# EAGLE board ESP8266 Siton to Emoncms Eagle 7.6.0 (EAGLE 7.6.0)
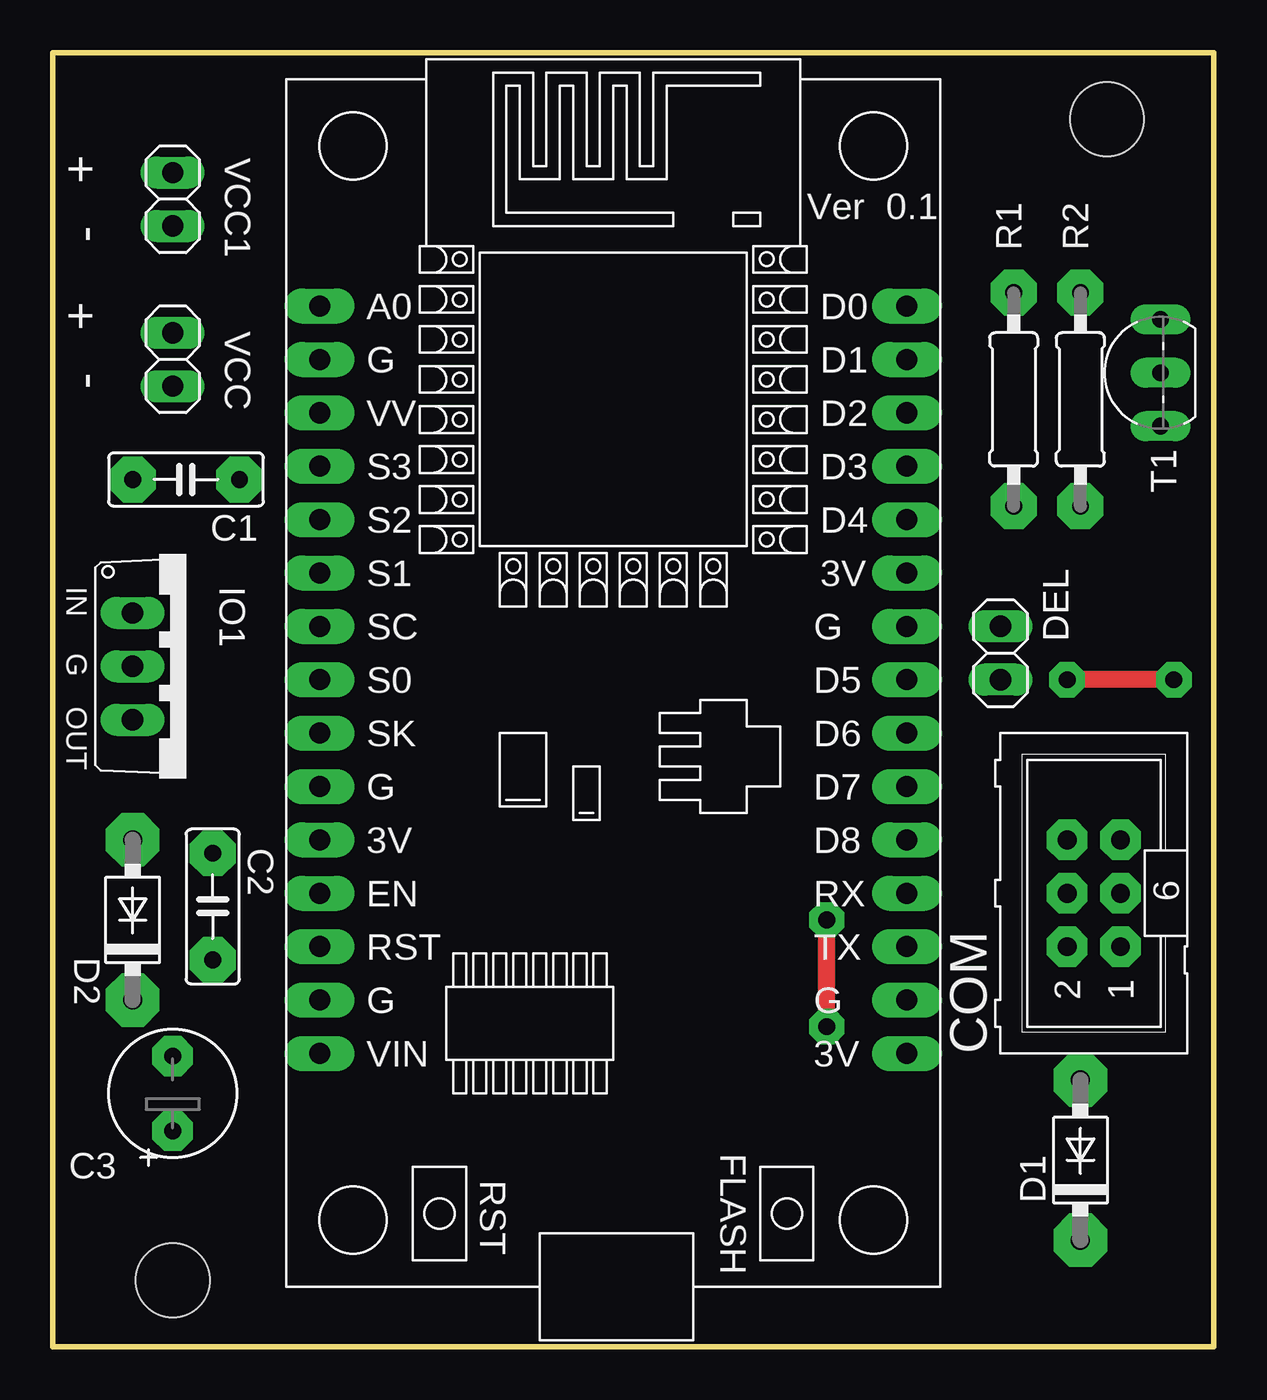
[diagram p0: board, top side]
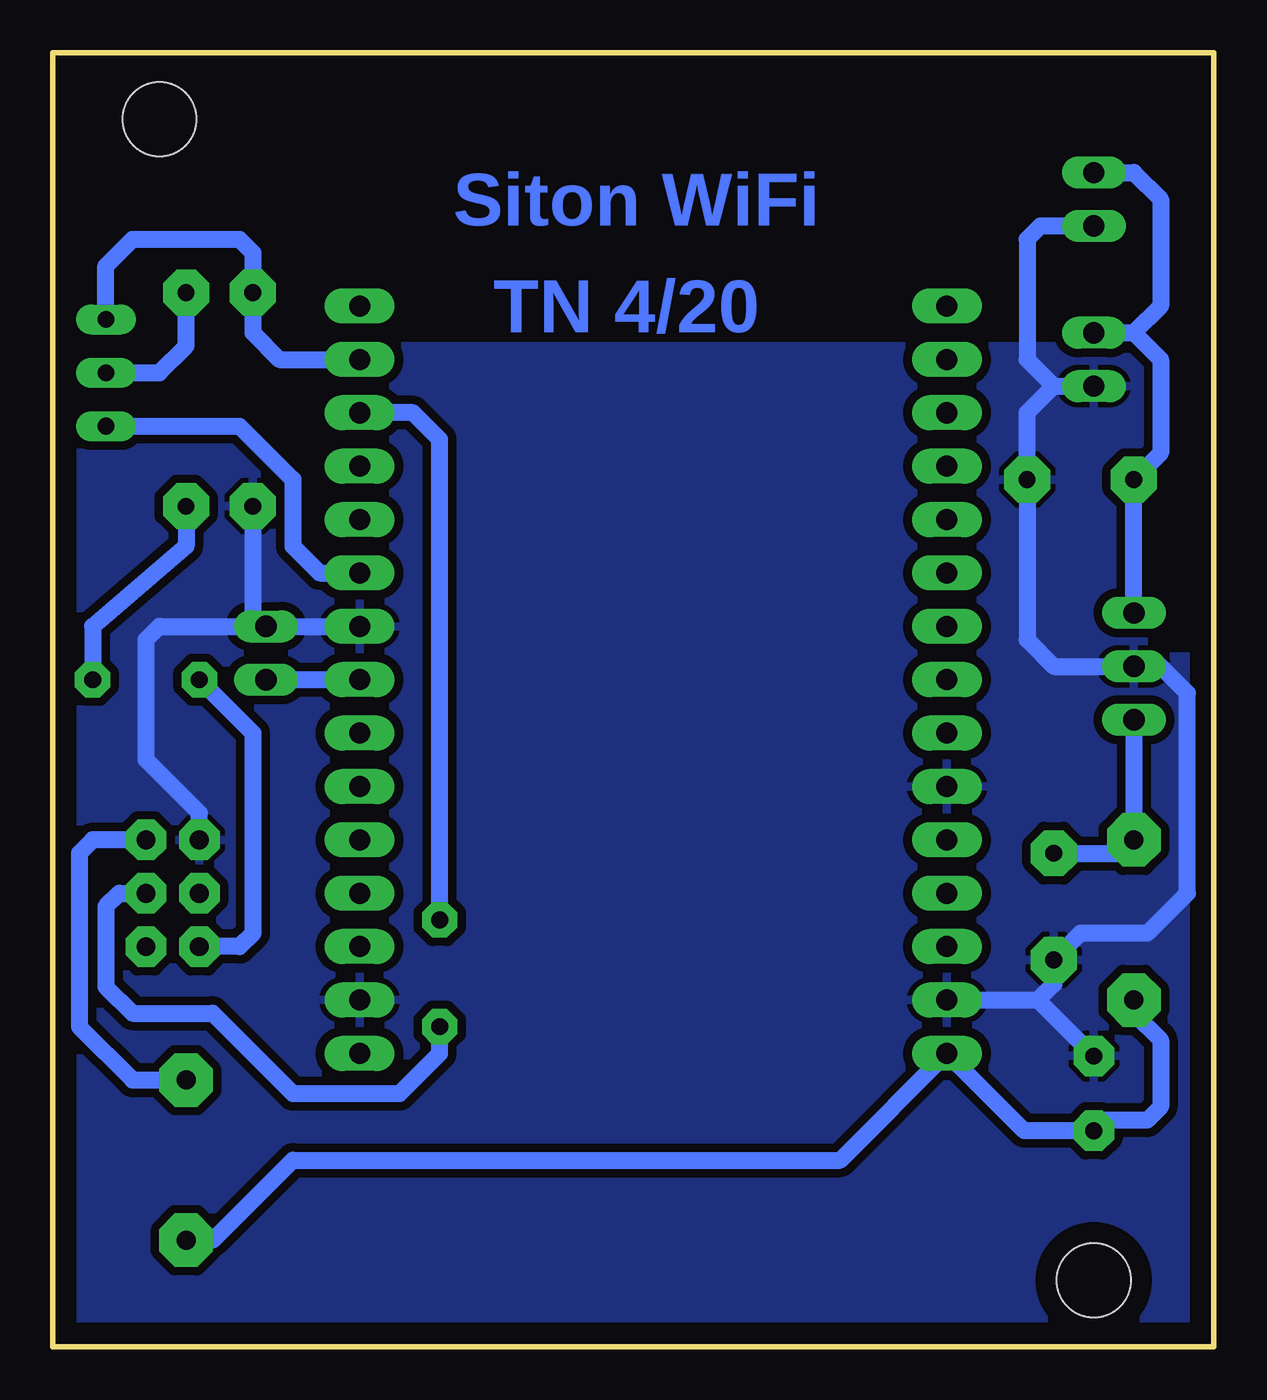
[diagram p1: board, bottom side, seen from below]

Size 55.24 x 61.59 mm. Coordinates in mm from the lower left corner, seen from the top.
Outline: 0,0 55.24,0 55.24,61.59 0,61.59 0,0
Copper layers (1*16): Top 0.035mm / dielectric 1.5mm / Bottom 0.035mm
Design rules "default": minimum track width 10mil, minimum drill 24mil, track to track 8mil, track to pad 8mil, pad to pad 8mil, via to via 8mil, smd to smd 8mil, copper to edge 40mil, drill to drill 8mil, minimum pad ring 10mil, minimum via ring 8mil, stop-mask expansion 4mil, vias tented up to drill 0mil, thermal gap 10mil
Holes 3.5 mm at 50.16,58.42 5.71,3.17
bRestrict: area 0,33.7 to 2.5,51.4

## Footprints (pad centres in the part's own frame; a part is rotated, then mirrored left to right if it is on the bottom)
C050-025X075 = drill 0.8 pad 2.184 octagon: 1 -2.54,0; 2 2.54,0
E3,5-8 = drill 0.8 pad 1.93 octagon: + -1.778,0; - 1.778,0
ML6 = drill 0.9 pad 1.93 octagon: 1 -2.54,-1.27; 2 -2.54,1.27; 3 0,-1.27; 4 0,1.27; 5 2.54,-1.27; 6 2.54,1.27
DO41-7 = drill 0.9 pad 2.54 octagon: A 3.81,0; C -3.81,0
1X02 = drill 1.016 long: 1 -1.27,0; 2 1.27,0
NODEMCU = drill 1 pad 1.676 long: 1 -13.97,17.78; 2 -13.97,15.24; 3 -13.97,12.7; 4 -13.97,10.16; 5 -13.97,7.62; 6 -13.97,5.08; 7 -13.97,2.54; 8 -13.97,0; 9 -13.97,-2.54; 10 -13.97,-5.08; 11 -13.97,-7.62; 12 -13.97,-10.16; 13 -13.97,-12.7; 14 -13.97,-15.24; 15 -13.97,-17.78; 16 13.97,-17.78; 17 13.97,-15.24; 18 13.97,-12.7; 19 13.97,-10.16; 20 13.97,-7.62; 21 13.97,-5.08; 22 13.97,-2.54; 23 13.97,0; 24 13.97,2.54; 25 13.97,5.08; 26 13.97,7.62; 27 13.97,10.16; 28 13.97,12.7; 29 13.97,15.24; 30 13.97,17.78
TO220V = drill 1.016 long: 1 -2.54,-2.54; 2 0,-2.54; 3 2.54,-2.54
0207/10 = drill 0.8 pad 2.184 octagon: 1 -5.08,0; 2 5.08,0
TO92-CBE = drill 0.8 pad 1.422 long: B 0,0; C -2.54,0; E 2.54,0

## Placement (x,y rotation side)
C1  100n  [C050-025X075]  6.35,41.27 180 top
C2  100n  [C050-025X075]  7.62,20.96 90 top
C3  220uF  [E3,5-8]  5.71,12.06 90 top
COM  [ML6]  49.53,21.59 90 top
D1  1N5819  [DO41-7]  48.9,8.89 90 top
D2  1N4007  [DO41-7]  3.81,20.32 90 top
DEL  [1X02]  45.09,33.02 90 top
E$1  [NODEMCU]  26.67,31.75 0 top
IO1  6V  [TO220V]  6.35,32.39 270 top
R1  1k  [0207/10]  45.72,45.08 90 top
R2  1k  [0207/10]  48.9,45.08 90 top
T1  BC337  [TO92-CBE]  52.71,46.36 90 top
VCC  [1X02]  5.71,46.99 270 top
VCC1  [1X02]  5.71,54.61 270 top

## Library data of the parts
C1-C3 COM D1 D2 R1 R2 T1 = 11moje
DEL VCC VCC1 = pinhead
E$1 = nodemcu
IO1 = linear

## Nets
GND: C1.1 C2.1 C3.- COM.6 E$1.10 E$1.14 E$1.17 E$1.24 IO1.2 R1.1 VCC1.2 VCC.2
S$1: COM.3 E$1.28
S$2: E$1.25 T1.C
S$3: R2.2 T1.B
S$4: COM.2 R2.1
S$6: COM.5 D1.A
S$7: E$1.29 R1.2 T1.E
S$8: C3.+ D1.C D2.C E$1.15
S$9: DEL.1 E$1.23
S$10: C2.2 D2.A IO1.3
S$12: C1.2 IO1.1 VCC1.1 VCC.1

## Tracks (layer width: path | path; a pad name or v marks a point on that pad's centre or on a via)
GND
  Bottom 0.813: E$1.14 8.38,16.51 | 8.38,16.51 C3.- | 7.62,45.72 8.89,44.45 C1.1 8.89,33.66 7.62,32.39 IO1.2 2.54,32.39 1.27,31.11 1.27,21.59 3.18,19.68 6.35,19.68 C2.1 7.62,17.27 8.38,16.51 | 7.62,45.72 VCC.2 | VCC1.2 8.26,53.34 8.89,52.7 8.89,46.99 7.62,45.72 | 45.72,34.29 E$1.24 | R1.1 45.72,34.29 | COM.6 48.26,25.4 50.8,27.94 50.8,33.66 50.16,34.29 45.72,34.29
  pour Bottom (isolate 0.406): 55.24,61.59 43.18,61.59 43.18,47.62 0,47.62 0,0 55.24,0
S$1  (via drill 0.8 pad 1.68)
  Top 0.813: v36.83,15.24 v36.83,20.32
  Bottom 0.813: E$1.28 38.1,44.45 36.83,43.18 v36.83,20.32 | COM.3 52.07,21.59 52.71,20.96 52.71,17.14 51.43,15.87 47.63,15.87 43.82,12.06 38.74,12.06 36.83,13.97 v36.83,15.24
S$2
  Bottom 0.813: T1.C 46.35,43.81 43.82,41.27 43.82,38.1 42.54,36.83 E$1.25
S$3
  Bottom 0.813: T1.B 50.16,46.36 48.9,47.62 R2.2
S$4  (via drill 0.8 pad 1.68)
  Top 0.813: v53.34,31.75 v48.26,31.75
  Bottom 0.813: R2.1 48.9,38.1 53.34,34.29 v53.34,31.75 | v48.26,31.75 45.72,29.21 45.72,19.68 46.35,19.05 COM.2
S$6
  Bottom 0.813: COM.5 53.34,24.13 53.98,23.5 53.98,15.24 51.43,12.7 D1.A
S$7
  Bottom 0.813: T1.E 52.71,51.43 51.43,52.7 46.35,52.7 45.72,52.07 R1.2 45.72,48.26 44.45,46.99 E$1.29
S$8
  Bottom 0.813: D2.C 3.81,15.87 2.54,14.6 2.54,11.43 3.18,10.79 5.21,10.79 C3.+ 9.02,10.29 E$1.15 17.78,8.89 43.82,8.89 47.63,5.08 D1.C
S$9
  Bottom 0.813: DEL.1 E$1.23
S$10
  Bottom 0.813: IO1.3 D2.A 4.45,23.5 C2.2
S$12
  Bottom 0.813: VCC.1 3.81,48.26 | 3.81,48.26 2.54,46.99 2.54,42.55 C1.2 IO1.1 | VCC1.1 3.81,55.88 2.54,54.61 2.54,49.53 3.81,48.26

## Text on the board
Bottom: Siton WiFi | TN 4/20
tNames: + | - | + | - | IN | G | OUT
